(* Generated automatically by TwinCAT - (read only) *)
VAR_CONFIG
	.LON_IN_1 AT %IB40 : ST_LON_Parameter_IN_36B;
	.LON_OUT_1 AT %QB40 : ST_LON_Parameter_OUT_36B;
	.LON_IN_2 AT %IB80 : ST_LON_Parameter_IN_36B;
	.LON_OUT_2 AT %QB80 : ST_LON_Parameter_OUT_36B;
	.LON_IN_3 AT %IB120 : ST_LON_Parameter_IN_36B;
	.LON_OUT_3 AT %QB120 : ST_LON_Parameter_OUT_36B;
	.LON_IN_4 AT %IB160 : ST_LON_Parameter_IN_36B;
	.LON_OUT_4 AT %QB160 : ST_LON_Parameter_OUT_36B;
	.LON_IN_5 AT %IB200 : ST_LON_Parameter_IN_36B;
	.LON_OUT_5 AT %QB200 : ST_LON_Parameter_OUT_36B;
	.LON_IN_6 AT %IB240 : ST_LON_Parameter_IN_36B;
	.LON_OUT_6 AT %QB240 : ST_LON_Parameter_OUT_36B;
	.LON_IN_7 AT %IB280 : ST_LON_Parameter_IN_36B;
	.LON_OUT_7 AT %QB280 : ST_LON_Parameter_OUT_36B;
END_VAR
